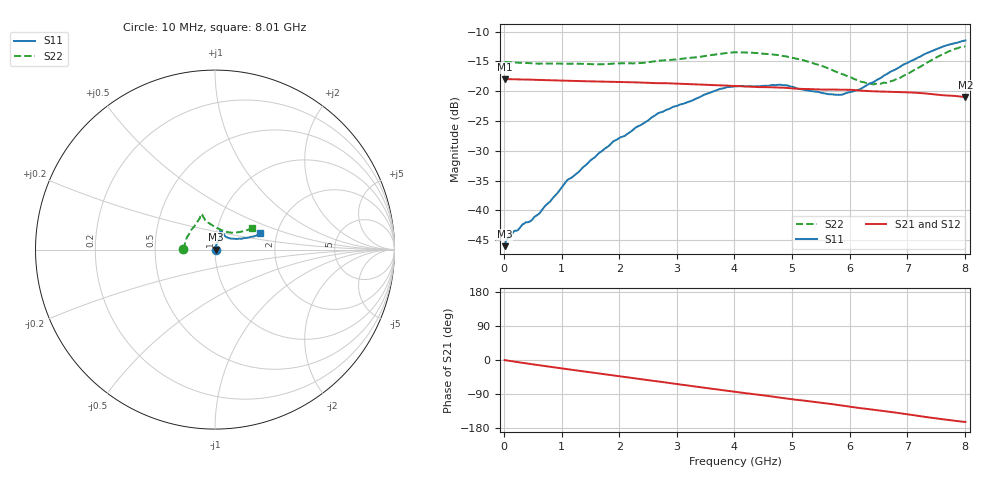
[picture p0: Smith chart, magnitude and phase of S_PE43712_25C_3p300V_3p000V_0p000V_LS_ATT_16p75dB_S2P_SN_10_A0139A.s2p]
! DEVICE ID: PE43712
! File Path: z:\PE43713\PE43713_CHAR_NOM_04292014\AMB\3p300\LS_ATT_16p75dB\PE43713_AMB_3p300V_3p000V_0p000V_LS_ATT_16p75dB_S2P_SN_10_A0139A.s2p
! Serial: 10
! Lot: A0139A
! Temp: 25C
! VDD: 3.300
! VSS: 0.000
! Control_Hi: 3.000
! Control_Lo: 0.000
! Attenuation Step: 16.75dB
! Port 1: RF1
! Port 2: RF2
! ThroughPath:1-2
! IDD: 0.0001461837
! ISS: -3.74e-008
#  Hz  S  RI  R  50
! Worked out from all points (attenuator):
!   801 points, 10 MHz to 8.01 GHz, reference 50 ohm
!   highest |S21| = -17.96 dB at 10 MHz (marker M1); lowest = -21.0 dB at 8.01 GHz (marker M2)
!   lowest |S11| = -46.0 dB at 10 MHz (marker M3), VSWR 1.01, Z = 50.5 + j0.0426 ohm
!   |S11| at or under -10 dB: start of sweep to end of sweep
!   |S22| runs from -18.8 to -12.5 dB; largest |S21 - S12| = 0.00047
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1e7  0.00499 0.000422  0.1264 -0.000655  0.1265 -0.000591  -0.1762 0.00116
1.6e8  0.00612 0.00238  0.1258 -0.00832  0.1258 -0.0083  -0.174 0.0111
6e8  0.00567 0.00739  0.121 -0.0293  0.121 -0.0293  -0.1668 0.0349
9.2e8  0.00476 0.013  0.1154 -0.0431  0.1155 -0.0431  -0.1626 0.0519
1.09e9  0.00477 0.0171  0.1118 -0.0498  0.1119 -0.0499  -0.1587 0.0615
1.35e9  0.00582 0.0217  0.106 -0.0596  0.106 -0.0596  -0.1528 0.0737
1.9e9  0.0115 0.0363  0.091 -0.0781  0.0909 -0.0781  -0.1353 0.104
2.11e9  0.014 0.0404  0.0843 -0.0844  0.0843 -0.0843  -0.1294 0.113
2.68e9  0.0254 0.0605  0.0642 -0.0976  0.0642 -0.0977  -0.1049 0.147
3.72e9  0.0318 0.0984  0.0233 -0.1097  0.0232 -0.1097  -0.0815 0.1882
4.01e9  0.0319 0.1051  0.0118 -0.1101  0.0118 -0.1101  -0.081 0.1963
4.79e9  0.0326 0.1088  -0.0171 -0.1059  -0.0172 -0.106  -0.0691 0.1878
5.35e9  0.0437 0.09  -0.0356 -0.0979  -0.0355 -0.0978  -0.0546 0.1645
5.64e9  0.0539 0.0775  -0.0441 -0.0935  -0.0441 -0.0935  -0.0368 0.15
5.87e9  0.0636 0.0689  -0.0517 -0.0892  -0.0516 -0.0892  -0.0186 0.1382
6.17e9  0.0822 0.0627  -0.0605 -0.0813  -0.0603 -0.0814  0.00995 0.1211
6.38e9  0.0999 0.0618  -0.0649 -0.076  -0.0648 -0.076  0.0332 0.1102
6.68e9  0.1298 0.0602  -0.0717 -0.0682  -0.0715 -0.0682  0.069 0.0977
6.99e9  0.1595 0.0637  -0.0783 -0.059  -0.0781 -0.0589  0.1014 0.094
7.37e9  0.1997 0.0712  -0.0836 -0.0456  -0.0835 -0.0455  0.1455 0.0999
7.72e9  0.2323 0.0798  -0.0854 -0.0341  -0.0853 -0.0342  0.1853 0.1113
8.01e9  0.2511 0.0903  -0.0857 -0.0254  -0.0855 -0.0256  0.2061 0.1187
